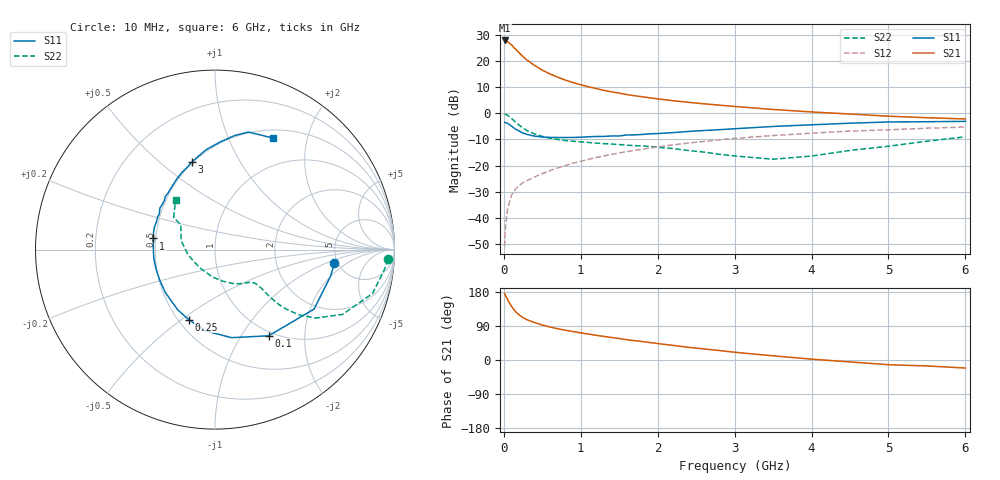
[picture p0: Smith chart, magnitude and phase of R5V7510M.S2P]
! SIEMENS Small Signal Semiconductors
! BFR183
! Si NPN RF Bipolar Junction Transistor in SOT23
! VCE = 0.75 V  IC = 10 mA
! Common Emitter S-Parameters:  May  1996
# GHz  S  MA  R  50
!  f  S11  S21  S12  S22
! GHz  MAG  ANG  MAG  ANG  MAG  ANG  MAG  ANG
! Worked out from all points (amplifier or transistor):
!   36 points, 10 MHz to 6 GHz, reference 50 ohm
!   highest |S21| = 27.8 dB at 10 MHz (marker M1)
!   |S21| within 3 dB of that: start of sweep to 141.1 MHz
!   unconditionally stable (mu >= 1): 660.9 MHz to 2.894 GHz
!   at 250 MHz: K = 0.65, MSG = 24.0 dB, |S12| = -26.5 dB
!   at 1.4 GHz: K = 1.08, MAG = 10.2 dB, |S12| = -15.7 dB
!   at 6 GHz: K = 0.95, MSG = 1.5 dB, |S12| = -5.3 dB
!   S11 on the Smith chart (normalised r, x): 10 MHz: 4.67, -1.28; 100 MHz: 0.94, -1.33; 250 MHz: 0.56, -0.53; 1 GHz: 0.49, +0.07; 3 GHz: 0.49, +0.65; 6 GHz: 0.60, +1.47
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0.01  0.6689 -6.5  24.48 175.8  0.0029 88.2  0.9647 -3.2
0.02  0.661 -12.9  24.34 171.0  0.0066 83.8  0.9523 -6.4
0.05  0.6437 -31.0  23.24 158.7  0.0152 75.1  0.9116 -15.5
0.1  0.5657 -58.1  20.15 141.4  0.0274 68.1  0.7978 -26.9
0.15  0.4992 -79.4  16.77 128.1  0.0355 60.7  0.6786 -34.2
0.2  0.4557 -96.7  14.13 118.9  0.0419 58.7  0.5906 -37.9
0.25  0.4168 -110.5  12.01 111.7  0.0473 57.5  0.5199 -39.8
0.3  0.3943 -121.9  10.38 106.3  0.0516 58.3  0.4684 -40.7
0.4  0.3656 -139.2  8.145 98.8  0.0609 58.8  0.4024 -40.8
0.5  0.3513 -151.6  6.623 92.3  0.0704 60.0  0.3607 -40.3
0.6  0.3457 -162.3  5.614 87.1  0.0804 60.9  0.3337 -39.8
0.7  0.3443 -171.3  4.872 82.5  0.0903 61.7  0.3159 -39.8
0.8  0.3434 -178.0  4.284 78.6  0.1004 61.9  0.3009 -39.8
1  0.3484 169.7  3.489 71.6  0.1211 61.6  0.284 -40.6
1.1  0.3548 164.9  3.2 68.4  0.1319 61.4  0.2766 -42.1
1.6  0.3844 143.0  2.265 53.6  0.1848 57.9  0.2449 -49.2
2.2  0.4263 124.0  1.728 38.6  0.2485 51.8  0.2113 -63.1
3  0.5054 104.8  1.346 20.5  0.3304 41.6  0.1528 -95.7
3.5  0.5587 95.1  1.179 11.0  0.3746 34.7  0.1324 -131.1
4.5  0.6447 80.3  0.965 -5.1  0.456 21.5  0.1951 165.2
5.5  0.6878 68.0  0.82 -15.7  0.5175 9.8  0.292 142.0
6  0.6995 62.7  0.777 -21.2  0.5449 2.3  0.3545 128.3
